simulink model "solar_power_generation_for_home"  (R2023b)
settings: Solver=VariableStepAuto  StartTime=0.0  StopTime=10.0  RelTol=1e-3
undefined symbols (not defined in the file or in its folder): bridge, full, phase, pulses, Single
libraries: spsSeriesRLCBranchLib x6, spsVoltageMeasurementLib x3, spsDiodeLib x1, spsIGBTDiodeLib x1, spsPVArrayLib x1, spsPWMGenerator2LevelLib x1, spsUniversalBridgeLib x1, sps_lib x1

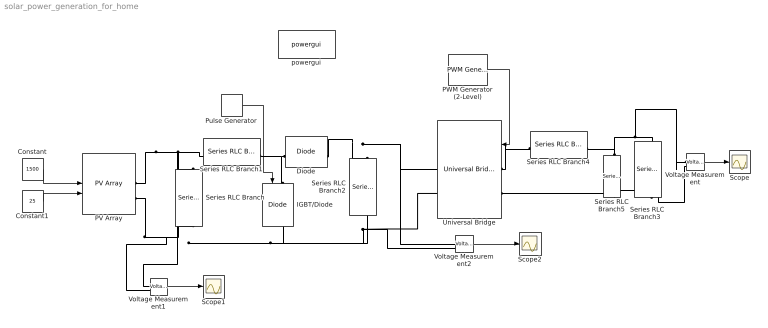
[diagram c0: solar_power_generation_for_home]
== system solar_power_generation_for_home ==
  Constant : Constant  Value=1500
  Constant1 : Constant  Value=25
  Diode : spsDiodeLib/Diode  Ron=0.001  Lon=0  Vf=0.8  IC=0  UseSnubber=0  Rs=500  Cs=250e-9  Measurements=on
  IGBT/Diode : spsIGBTDiodeLib/IGBT//Diode  Ron=1e-3  Rs=1e5  Cs=inf  Measurements=on
  PV Array : spsPVArrayLib/PV Array  Npar=20  Nser=5  PlotType=array @ 1000 W/m2 & specified temperatures  S_vec="[ 1000  500  100 ]"  Temp_C_vec="[ 45 25  ]"  ModuleName=User-defined  PlotWhenSelected=off  Pm=213.15  Ncell=60  Voc=36.3  Isc=7.84  Vm=29  Im=7.35  beta_Voc_pc=-0.36099  alpha_Isc_pc=0.102  beta_Voc=-0.13104  alpha_Isc=0.0079968  IL=7.8654  I0=2.9273e-10  nI=0.98119  Rsh=313.0553  Rs=0.39381  RobustModel=off  RobustCellTemperature=313.3991  BAL=on  Tc=1e-6  Tfilter=5e-5
  PWM Generator (2-Level) : spsPWMGenerator2LevelLib/PWM Generator (2-Level)  ModulatorType=Single-phase full-bridge (4 pulses)  ModulatorMode=Unsynchronized  Fc=27*60  Pc=90  nF=27  MinMax="[ -1  1 ]"  SamplingTechnique=Natural  ModulatingSignals=on  m=0.8  Freq=60  Phase=0  Ts=0  ShowCarrierOutport=off
  Pulse Generator : DiscretePulseGenerator  PulseType=Time based  Period=1/1500  PulseWidth=50
  Scope : Scope
  Scope1 : Scope
  Scope2 : Scope
  Series RLC Branch : spsSeriesRLCBranchLib/Series RLC Branch  LConnTagsString=__new0  RConnTagsString=__new0  BranchType=C  Resistance=1  Inductance=1e-3  SetiL0=off  InitialCurrent=0  Capacitance=0.006  Setx0=off  InitialVoltage=0  Measurements=None
  Series RLC Branch1 : spsSeriesRLCBranchLib/Series RLC Branch  LConnTagsString=__new0  RConnTagsString=__new0  BranchType=L  Resistance=1  Inductance=0.02  SetiL0=off  InitialCurrent=0  Capacitance=0.006  Setx0=off  InitialVoltage=0  Measurements=None
  Series RLC Branch2 : spsSeriesRLCBranchLib/Series RLC Branch  LConnTagsString=__new0  RConnTagsString=__new0  BranchType=C  Resistance=1  Inductance=1e-3  SetiL0=off  InitialCurrent=0  Capacitance=0.006  Setx0=off  InitialVoltage=0  Measurements=None
  Series RLC Branch3 : spsSeriesRLCBranchLib/Series RLC Branch  LConnTagsString=__new0  RConnTagsString=__new0  BranchType=R  Resistance=1  Inductance=1e-3  SetiL0=off  InitialCurrent=0  Capacitance=0.006  Setx0=off  InitialVoltage=0  Measurements=None
  Series RLC Branch4 : spsSeriesRLCBranchLib/Series RLC Branch  LConnTagsString=__new0  RConnTagsString=__new0  BranchType=L  Resistance=1  Inductance=0.02  SetiL0=off  InitialCurrent=0  Capacitance=0.006  Setx0=off  InitialVoltage=0  Measurements=None
  Series RLC Branch5 : spsSeriesRLCBranchLib/Series RLC Branch  LConnTagsString=__new0  RConnTagsString=__new0  BranchType=C  Resistance=1  Inductance=1e-3  SetiL0=off  InitialCurrent=0  Capacitance=0.006  Setx0=off  InitialVoltage=0  Measurements=None
  Universal Bridge : spsUniversalBridgeLib/Universal Bridge  Arms=2  SnubberResistance=1e5  SnubberCapacitance=inf  Device=IGBT / Diodes  Ron=1e-3  Lon=0  ForwardVoltages="[  0  0  ]"  ForwardVoltage=0  GTOparameters=[ 10e-6 , 20e-6 ]  IGBTparameters=[ 1e-6 , 2e-6 ]  Measurements=None  Measurements_2=None  converterType=Rectifier
  Voltage Measurement : spsVoltageMeasurementLib/Voltage Measurement  PhasorSimulation=off  OutputType=Complex  PSBequivalent=0
  Voltage Measurement1 : spsVoltageMeasurementLib/Voltage Measurement  PhasorSimulation=off  OutputType=Complex  PSBequivalent=0
  Voltage Measurement2 : spsVoltageMeasurementLib/Voltage Measurement  PhasorSimulation=off  OutputType=Complex  PSBequivalent=0
  powergui : sps_lib/powergui  Priority=1  SimulationMode=Continuous  SampleTime=50e-6  frequency=60  Iterations=50  frequencyindice=0  Pbase=100e6  ErrMax=1e-4  UnitsV=kV  UnitsW=MW  buscounter=0  FunctionMessages=off  echomessages=off  EnableUseOfTLC=off  CurrentSourceSwitches=off  DisableSnubberDevices=off  DisableRonSwitches=off  DisableVfSwitches=off  DisplayEquations=off  AutomaticDiscreteSolvers=off  SolverType=Tustin/Backward Euler (TBE)  Interpol=off  ExternalGateDelay=off  methode=off  Ts=100  x0status=blocks  SPID=on  SwTol=0  HookPort=off  NonlinearTolerance=1e-4  nMaxIteration=100  ContinueOnMaxIteration=off  RestoreLinks=warning  ResistiveCurrentMeasurement=off  Frange=[0:2:500]  Ylog=off  Xlog=on  ShowGrid=off  save=off  variable=ZData  structure=0  ZoomFFT=off  StartTime=0.0  cycles=1  DisplayStyle=1  fundamental=60  FreqAxis=off  MaxFrequency=1000  frequencyindicesteady=1  RmsSteady=1  display=off
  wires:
  Constant/1 -> PV Array/1
  Constant1/1 -> PV Array/2
  PWM Generator (2-Level)/1 -> Universal Bridge/1
  Voltage Measurement/1 -> Scope/1
  Pulse Generator/1 -> IGBT/Diode/1
  Voltage Measurement1/1 -> Scope1/1
  Voltage Measurement2/1 -> Scope2/1
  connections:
  PV Array/RConn1 -- Voltage Measurement1/LConn1 -- Series RLC Branch1/RConn1 -- Series RLC Branch/LConn1
  PV Array/RConn2 -- Voltage Measurement1/LConn2 -- Universal Bridge/RConn2 -- Voltage Measurement2/LConn2 -- Series RLC Branch2/RConn1 -- IGBT/Diode/RConn1 -- Series RLC Branch/RConn1
  Diode/LConn1 -- Series RLC Branch1/LConn1 -- IGBT/Diode/LConn1
  Diode/RConn1 -- Universal Bridge/RConn1 -- Voltage Measurement2/LConn1 -- Series RLC Branch2/LConn1
  Series RLC Branch5/LConn1 -- Series RLC Branch3/LConn1 -- Voltage Measurement/LConn1 -- Series RLC Branch4/LConn1
  Series RLC Branch3/RConn1 -- Voltage Measurement/LConn2 -- Series RLC Branch5/RConn1 -- Universal Bridge/LConn2
  Universal Bridge/LConn1 -- Series RLC Branch4/RConn1
